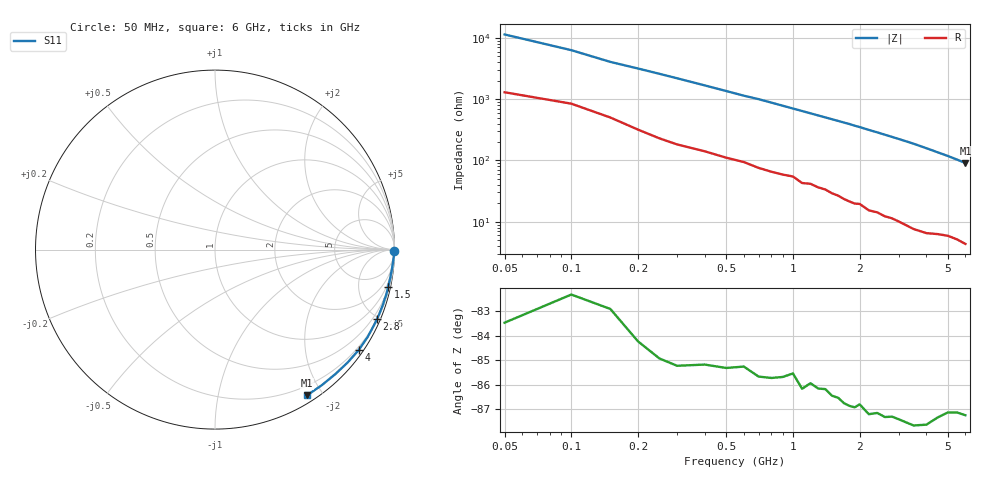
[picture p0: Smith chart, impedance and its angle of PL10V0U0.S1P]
! Infineon Technologies  Discrete & RF Semiconductors
! BAR 64-04W /-05W /-06W
! Si PIN Diode in SOT323
! VR = 10 V
! S-Parameters:  October  2008
# GHz  S  MA  R  50
!  f  S11
! GHz  MAG  ANG
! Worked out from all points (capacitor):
!   34 points, 50 MHz to 6 GHz, reference 50 ohm
!   read as one part to ground: C = 263 fF near 50 MHz
!   lowest |Z| = 90.7 ohm at 6 GHz (marker M1)
!   S11 on the Smith chart (normalised r, x): 50 MHz: open; 1.5 GHz: 0.58, -9.40; 2.8 GHz: 0.23, -4.84; 4 GHz: 0.13, -3.17; 6 GHz: 0.09, -1.81
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0.05  0.999 -0.5
0.1  0.9979 -0.9
0.15  0.997 -1.4
0.3  0.9962 -2.6
0.4  0.995 -3.4
0.6  0.9928 -5.0
0.7  0.9925 -5.7
0.8  0.9916 -6.5
1  0.9891 -8.1
1.1  0.9897 -8.9
1.2  0.9881 -9.7
1.5  0.9871 -12.1
1.6  0.9866 -12.9
1.7  0.9867 -13.7
1.8  0.9864 -14.5
1.9  0.9859 -15.4
2  0.9846 -16.2
2.2  0.9851 -18.0
2.4  0.9834 -19.7
2.6  0.9831 -21.5
2.8  0.9816 -23.3
3  0.9811 -25.1
3.5  0.98 -29.8
4  0.9767 -35.0
4.5  0.9704 -40.4
5  0.9649 -45.8
5.5  0.9617 -51.6
6  0.9603 -57.7
